FUNCTION_BLOCK FB 1
TITLE =
//Erste_Schritte_AWL
AUTHOR : Siemens
FAMILY : GetStart
NAME : ENGINE
VERSION : 1.0


VAR_INPUT
  Switch_On : BOOL ;	//Motor einschalten
  Switch_Off : BOOL ;	//Motor ausschalten
  Failure : BOOL ;	//Motorstörung, führt zum Ausschalten
  Actual_Speed : INT ;	//tatsächliche Motordrehzahl
END_VAR
VAR_OUTPUT
  Engine_On : BOOL ;	//Motor wird eingeschaltet
  Preset_Speed_Reached : BOOL ;	//Solldrehzahl erreicht
END_VAR
VAR
  Preset_Speed : INT  := 1500;	//geforderte Motordrehzahl
END_VAR
BEGIN
NETWORK
TITLE =Motor einschalten, Negation von Signalen
//Zum Einschalten des Motors werden die Operationen S (Setzen) und R (Rücksetzen)
//verwendet und so ein speicherndes Verhalten erreicht.
//
//Der Motor wird eingeschaltet, wenn die Variable #Switch_On eingeschaltet ist
//(Signalzustand "1" führt) und die Variable "Automatikbetrieb" ausgeschaltet ist
//(Signalzustand "0" führt). Die Abfrage auf Signalzustand "0" wird durch ein
//nachgestelltes "N" also "UN" dargestellt.
//
//Der Motor wird wieder ausgeschaltet, wenn die Variable #Switch_Off einge-
//schaltet ist oder die Variable #Failure Signalzustand "0" führt. #Failure
//ist ein "nullaktives" Signal, das im Normalfall "1" führt (wenn keine Störung
//ansteht) und im Störfall "0" führt. Auch hier erreichen wir die gewünschte
//Funktionalität, wenn wir das Signal #Failure mit "ON" auf Signalzustand "0"
//abfragen.
//
//Hinweis: "Bausteinlokale" Variablen werden mit #name dargestellt; sie sind nur
//im Baustein "gültig". Globale Variablen "name" stehen in Anführungszeichen; sie
//sind im gesamten Programm "gültig".
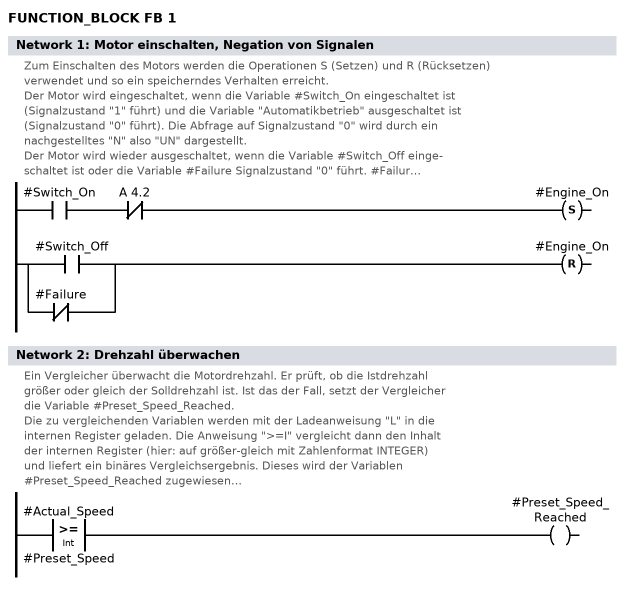
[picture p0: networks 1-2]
      U     #Switch_On;
      UN    A      4.2;
      S     #Engine_On;
      O     #Switch_Off;
      ON    #Failure;
      R     #Engine_On;
NETWORK
TITLE =Drehzahl überwachen
//Ein Vergleicher überwacht die Motordrehzahl. Er prüft, ob die Istdrehzahl
//größer oder gleich der Solldrehzahl ist. Ist das der Fall, setzt der Vergleicher
//die Variable #Preset_Speed_Reached.
//
//Die zu vergleichenden Variablen werden mit der Ladeanweisung "L" in die
//internen Register geladen. Die Anweisung ">=I" vergleicht dann den Inhalt
//der internen Register (hier: auf größer-gleich mit Zahlenformat INTEGER)
//und liefert ein binäres Vergleichsergebnis. Dieses wird der Variablen
//#Preset_Speed_Reached zugewiesen.
//
//Die Motor-Istdrehzahl ist ein Eingangs-Bausteinparameter (Deklaration "in"),
//da sie motorspezifisch ist. Auch die Solldrehzahl ist motorspezifisch; da sie
//jedoch ein fester Wert ist, kann sie statisch in den Motordaten gespeichert
//werden (Deklaration "stat"). Man spricht hier von "statischen Lokalvariablen".
      L     #Actual_Speed;
      L     #Preset_Speed;
      >=I   ;
      =     #Preset_Speed_Reached;
END_FUNCTION_BLOCK

DATA_BLOCK DB 1
TITLE =
//Erste_Schritte_AWL
AUTHOR : Siemens
FAMILY : GetStart
NAME : Petrol
VERSION : 1.0

 FB 1
BEGIN
   Switch_On := FALSE;
   Switch_Off := FALSE;
   Failure := FALSE;
   Actual_Speed := 0;
   Engine_On := FALSE;
   Preset_Speed_Reached := FALSE;
   Preset_Speed := 1500;
END_DATA_BLOCK

DATA_BLOCK DB 2
TITLE =
//Erste_Schritte_AWL
AUTHOR : Siemens
FAMILY : GetStart
NAME : Diesel
VERSION : 1.0

 FB 1
BEGIN
   Switch_On := FALSE;
   Switch_Off := FALSE;
   Failure := FALSE;
   Actual_Speed := 0;
   Engine_On := FALSE;
   Preset_Speed_Reached := FALSE;
   Preset_Speed := 1200;
END_DATA_BLOCK

FUNCTION FC 1: VOID
TITLE =
//Erste_Schritte_AWL
AUTHOR : Siemens
FAMILY : GetStart
NAME : FAN
VERSION : 1.0


VAR_INPUT
  Engine_On : BOOL ;	//Signal für das Einschalten des Motors
  Timer_Function : TIMER ;	//verwendete Zeitfunktion für die Ausschaltverzögerung
END_VAR
VAR_OUTPUT
  Fan_On : BOOL ;	//Signal für das Einschaltes des Lüfters
END_VAR
BEGIN
NETWORK
TITLE =Lüftersteuerung
//Mit dem Eingangsparameter #Engine_On wird über die Anweisung SA (Starte Zeit
//als Ausschaltverzögerung) die Variable #Timer_Function gestartet.
//#Timer_Function, mit dem Datentyp TIMER, steht hier für eine Zeitfunktion, die
//später beim Aufruf im OB 1 mit einem Zeitoperanden (z.B. T 1) versorgt wird.
//Für jedes Motor-Lüfter-Paar müssen Sie beim Aufruf einen anderen Zeitoperanden
//wählen.
//
//Vor dem Laden wird eine konstante Ausschaltverzögerung mit 4 s Dauer geladen.
//Sie können die Zeitdauer auch als Eingangsparameter mit dem Datentyp S5TIME
//übergeben, so daß für jeden Motor eine andere Nachlaufzeit für den jeweiligen
//Lüfter parametriert werden kann.
      U     #Engine_On;
      L     S5T#4S;
      SA    #Timer_Function;

      U     #Timer_Function;
      =     #Fan_On;
END_FUNCTION

ORGANIZATION_BLOCK OB 1
TITLE =
//Erste_Schritte_AWL
AUTHOR : Siemens
FAMILY : GetStart
NAME : Cycle
VERSION : 1.0


VAR_TEMP
  OB1_EV_CLASS : BYTE ;	//Bits 0-3 = 1 (Coming event), Bits 4-7 = 1 (Event class 1)
  OB1_SCAN_1 : BYTE ;	//1 (Cold restart scan 1 of OB 1), 3 (Scan 2-n of OB 1)
  OB1_PRIORITY : BYTE ;	//1 (Priority of 1 is lowest)
  OB1_OB_NUMBR : BYTE ;	//1 (Organization block 1, OB1)
  OB1_RESERVED_1 : BYTE ;	//Reserved for system
  OB1_RESERVED_2 : BYTE ;	//Reserved for system
  OB1_PREV_CYCLE : INT ;	//Cycle time of previous OB1 scan (milliseconds)
  OB1_MIN_CYCLE : INT ;	//Minimum cycle time of OB1 (milliseconds)
  OB1_MAX_CYCLE : INT ;	//Maximum cycle time of OB1 (milliseconds)
  OB1_DATE_TIME : DATE_AND_TIME ;	//Date and time OB1 started
END_VAR
BEGIN
NETWORK
TITLE =UND-Abfrage
//Wenn der "Taster 1" (E 0.1) und der "Taster 2" (E 0.2) eingeschaltet sind
//(d.h. Signalzustand "1" = 24V führen), dann ist die "Lampe Grün" (A 4.0)
//eingeschaltet.
//
//Es müssen beide Eingänge eingeschaltet sein, damit die Lampe leuchtet.
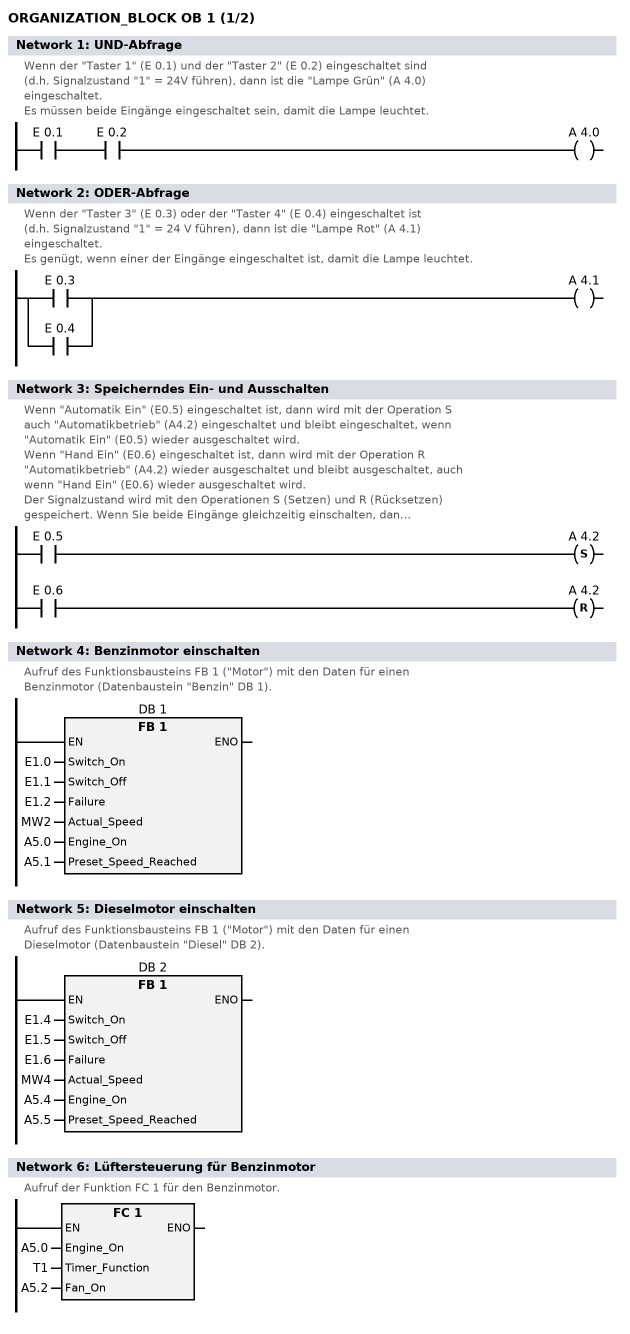
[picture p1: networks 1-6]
      U     E      0.1;
      U     E      0.2;
      =     A      4.0;

NETWORK
TITLE =ODER-Abfrage
//Wenn der "Taster 3" (E 0.3) oder der "Taster 4" (E 0.4) eingeschaltet ist
//(d.h. Signalzustand "1" = 24 V führen), dann ist die "Lampe Rot" (A 4.1)
//eingeschaltet.
//
//Es genügt, wenn einer der Eingänge eingeschaltet ist, damit die Lampe leuchtet.
      O     E      0.3;
      O     E      0.4;
      =     A      4.1;

NETWORK
TITLE =Speicherndes Ein- und Ausschalten
//Wenn "Automatik Ein" (E0.5) eingeschaltet ist, dann wird mit der Operation S
//auch "Automatikbetrieb" (A4.2) eingeschaltet und bleibt eingeschaltet, wenn
//"Automatik Ein" (E0.5) wieder ausgeschaltet wird.
//
//Wenn "Hand Ein" (E0.6) eingeschaltet ist, dann wird mit der Operation R
//"Automatikbetrieb" (A4.2) wieder ausgeschaltet und bleibt ausgeschaltet, auch
//wenn "Hand Ein" (E0.6) wieder ausgeschaltet wird.
//
//Der Signalzustand wird mit den Operationen S (Setzen) und R (Rücksetzen)
//gespeichert. Wenn Sie beide Eingänge gleichzeitig einschalten, dann
//wird zuerst das Setzen und dann das Rücksetzen bearbeitet. Bedingt durch
//die Programmierreihenfolge "siegt" letztendlich das Rücksetzen:
//"Automatik Ein" (A4.2) wird oder bleibt ausgeschaltet.
//Man sagt: "Rücksetzen hat Vorrang".
      U     E      0.5;
      S     A      4.2;
      U     E      0.6;
      R     A      4.2;


NETWORK
TITLE =Benzinmotor einschalten
//Aufruf des Funktionsbausteins FB 1 ("Motor") mit den Daten für einen
//Benzinmotor (Datenbaustein "Benzin" DB 1).
      CALL FB     1 , DB     1 (
           Switch_On                := E1.0,
           Switch_Off               := E1.1,
           Failure                  := E1.2,
           Actual_Speed             := MW2,
           Engine_On                := A5.0,
           Preset_Speed_Reached     := A5.1);


NETWORK
TITLE =Dieselmotor einschalten
//Aufruf des Funktionsbausteins FB 1 ("Motor") mit den Daten für einen
//Dieselmotor (Datenbaustein "Diesel" DB 2).
      CALL FB     1 , DB     2 (
           Switch_On                := E1.4,
           Switch_Off               := E1.5,
           Failure                  := E1.6,
           Actual_Speed             := MW4,
           Engine_On                := A5.4,
           Preset_Speed_Reached     := A5.5);


NETWORK
TITLE =Lüftersteuerung für Benzinmotor
//Aufruf der Funktion FC 1 für den Benzinmotor.
      CALL FC     1 (
           Engine_On                := A5.0,
           Timer_Function           := T1,
           Fan_On                   := A5.2);



NETWORK
TITLE =Lüftersteuerung für Dieselmotor
//Aufruf der Funktion FC 1 für den Dieselmotor.
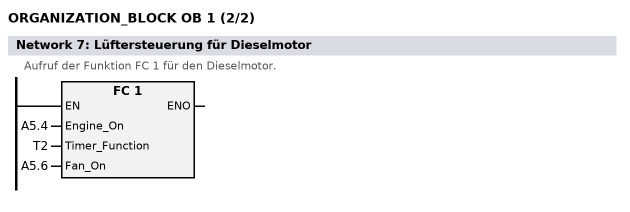
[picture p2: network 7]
      CALL FC     1 (
           Engine_On                := A5.4,
           Timer_Function           := T2,
           Fan_On                   := A5.6);



END_ORGANIZATION_BLOCK

